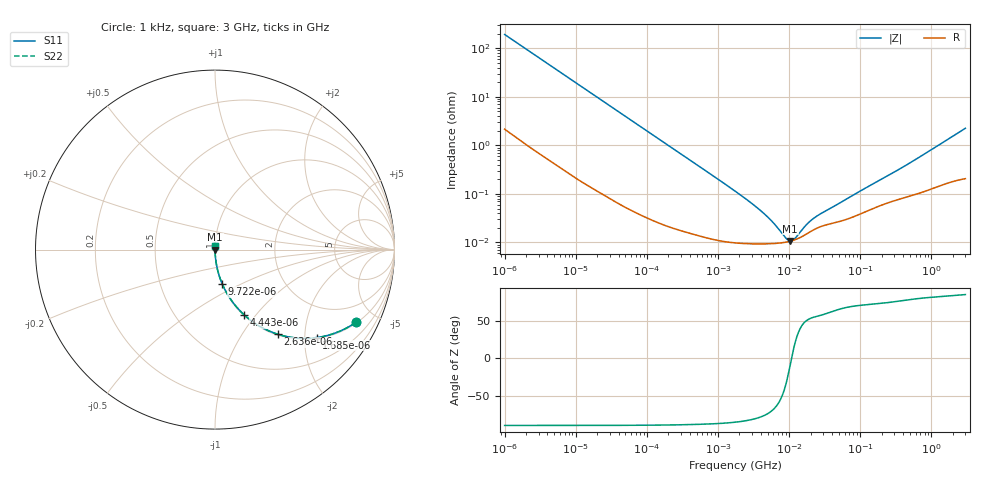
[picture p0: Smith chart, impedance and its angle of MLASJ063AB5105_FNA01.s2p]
! MLASJ063AB5105_FNA01  S-PARAMETER MODEL  ( Standard Model )
! Model Generated by TAIYO YUDEN Corporation (http://www.ty-top.com)
! Version 3.0
! TAIYO YUDEN Control No. 240422
! Copyright(c) 2012 TAIYO YUDEN CO.,LTD. All Rights Reserved.
! Product Description (link to TY-COMPAS)
! https://ds.yuden.co.jp/TYCOMPAS/or/detail?pn=MLASJ063AB5105KFNA01&u=M
! Products Name : Multilayer Ceramic Capacitors
! Characteristics :
!  Capacitance : 1 [uF] , Rated Voltage : 6.3 [V] , TCC : X5R
!  Case Size : 0.6 x 0.3 / 0.024 x 0.012 [mm/inch] , Thickness : 0.3 / 0.012 [mm/inch]
!  (Conditions: Temperature = 25 [degC] , DC Bias Voltage = 0 [V])
! External Node Assignments :
!  1  o---| |---o  2
! GND o---------o GND
! Frequency Range : 1kHz  -  3GHz  [ 401 STEP ]
# MHZ S RI R 50
! Freq[MHz].  S11 Real  S11 Imag  S21 Real  S21 Imag  S12 Real  S12 Imag  S22 Real  S22 Imag
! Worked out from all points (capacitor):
!   401 points, 1 kHz to 3 GHz, reference 50 ohm
!   read as one part in series: C = 827 nF near 1.077 kHz
!   lowest |Z| = 10.7 mohm at 10.37 MHz (marker M1)
!   series resonance near 10.81 MHz, so ESL is about 260 pH
!   S11 on the Smith chart (normalised r, x): 1 kHz: 1.04, -3.84; 1.685 kHz: 1.02, -2.29; 2.636 kHz: 1.02, -1.47; 4.443 kHz: 1.01, -0.87; 9.722 kHz: 1.00, -0.40; 3 GHz: 1.00, +0.04
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0.001  0.7841 -0.4059  0.2159 0.4059  0.2159 0.4059  0.7841 -0.4059
0.001251  0.7008 -0.4524  0.2992 0.4524  0.2992 0.4524  0.7008 -0.4524
0.001685  0.566 -0.4902  0.434 0.4902  0.434 0.4902  0.566 -0.4902
0.002636  0.3512 -0.472  0.6488 0.472  0.6488 0.472  0.3512 -0.472
0.004443  0.1627 -0.3638  0.8373 0.3638  0.8373 0.3638  0.1627 -0.3638
0.006451  0.0858 -0.2747  0.9142 0.2747  0.9142 0.2747  0.0858 -0.2747
0.009722  0.0406 -0.192  0.9594 0.192  0.9594 0.192  0.0406 -0.192
0.01216  0.0268 -0.156  0.9732 0.156  0.9732 0.156  0.0268 -0.156
0.033275  0.0042 -0.0588  0.9958 0.0588  0.9958 0.0588  0.0042 -0.0588
0.147855  0.000431 -0.0134  0.9996 0.0134  0.9996 0.0134  0.000431 -0.0134
1.732051  9.93e-05 -0.00114  0.9999 0.00114  0.9999 0.00114  9.93e-05 -0.00114
2.919173  9.42e-05 -0.000645  0.9999 0.000645  0.9999 0.000645  9.42e-05 -0.000645
4.399271  9.36e-05 -0.000386  0.9999 0.000386  0.9999 0.000386  9.36e-05 -0.000386
6.153411  9.52e-05 -0.000224  0.9999 0.000224  0.9999 0.000224  9.52e-05 -0.000224
8.933959  0.000101 -7.24e-05  0.9999 7.24e-05  0.9999 7.24e-05  0.000101 -7.24e-05
10.37087  0.000106 -1.56e-05  0.9999 1.56e-05  0.9999 1.56e-05  0.000106 -1.56e-05
12.03889  0.000114 4.05e-05  0.9999 -4.05e-05  0.9999 -4.05e-05  0.000114 4.05e-05
16.83921  0.000144 0.000165  0.9999 -0.000165  0.9999 -0.000165  0.000144 0.000165
21.06097  0.000175 0.000241  0.9998 -0.000241  0.9998 -0.000241  0.000175 0.000241
28.38055  0.000215 0.000336  0.9998 -0.000336  0.9998 -0.000336  0.000215 0.000336
256.0921  0.000675 0.00238  0.9993 -0.00238  0.9993 -0.00238  0.000675 0.00238
3000  0.00256 0.0223  0.9974 -0.0223  0.9974 -0.0223  0.00256 0.0223
